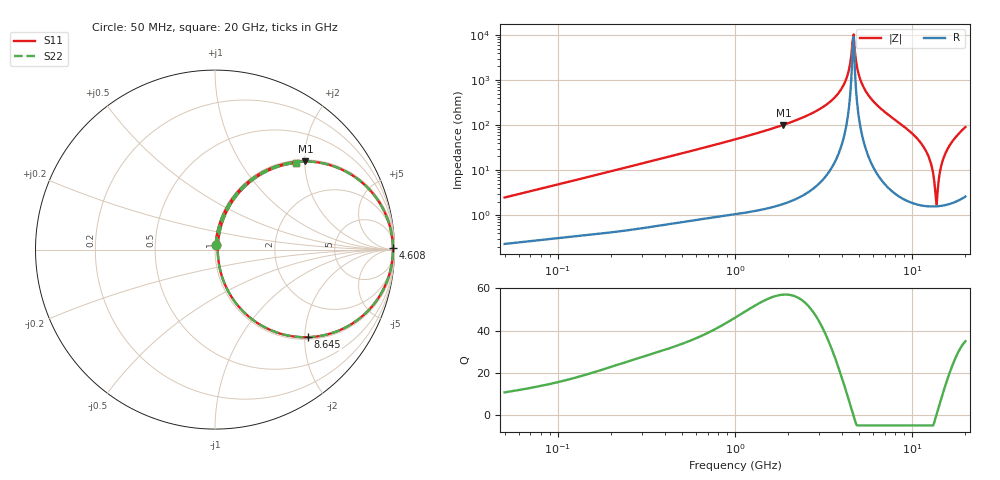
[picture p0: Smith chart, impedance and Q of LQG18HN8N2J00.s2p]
!Murata Part Number: LQG18HN8N2J00
!These Parameters are Measured in Series Mode Connection
!  o--[Z]--o
!Port1  Port2
!  o-------o
!Freq. Start=50[MHz] Stop=20[GHz], 401[Steps]
# Hz S RI R 50
!Freq.(Hz) S11(Real) S11(Imag) S21(Real) S21(Imag) S12(Real) S12(Imag) S22(Real) S22(Imag)
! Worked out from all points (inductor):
!   401 points, 50 MHz to 20 GHz, reference 50 ohm
!   read as one part in series: L = 7.7 nH near 51.52 MHz
!   highest Q = 57.1 at 1.876 GHz (marker M1), where L = 8.55 nH
!   self-resonance near 4.608 GHz
!   S11 on the Smith chart (normalised r, x): 50 MHz: 1.00, +0.05; 4.608 GHz: open; 8.645 GHz: 1.05, -2.08; 20 GHz: 1.05, +1.80
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5e7  0.00287 0.0243  0.9971 -0.0243  0.9971 -0.0243  0.00287 0.0243
1.364002e8  0.0076 0.0639  0.9924 -0.0639  0.9924 -0.0639  0.0076 0.0639
3.721004e8  0.0347 0.1672  0.9653 -0.1672  0.9653 -0.1672  0.0347 0.1672
1e9  0.1919 0.3831  0.8081 -0.3831  0.8081 -0.3831  0.1919 0.3831
1.875929e9  0.5037 0.4913  0.4963 -0.4913  0.4963 -0.4913  0.5037 0.4913
2.728004e9  0.7661 0.4133  0.2339 -0.4133  0.2339 -0.4133  0.7661 0.4133
3.415248e9  0.904 0.2802  0.096 -0.2802  0.096 -0.2802  0.904 0.2802
3.967106e9  0.9662 0.1562  0.0338 -0.1562  0.0338 -0.1562  0.9662 0.1562
4.34015e9  0.9864 0.071  0.0136 -0.071  0.0136 -0.071  0.9864 0.071
4.608136e9  0.9914 0.0108  0.00861 -0.0108  0.00861 -0.0108  0.9914 0.0108
4.748272e9  0.9911 -0.02  0.00895 0.02  0.00895 0.02  0.9911 -0.02
5.041459e9  0.9844 -0.0824  0.0156 0.0824  0.0156 0.0824  0.9844 -0.0824
5.433528e9  0.9641 -0.1608  0.0359 0.1608  0.0359 0.1608  0.9641 -0.1608
7.442007e9  0.7197 -0.4376  0.2803 0.4376  0.2803 0.4376  0.7197 -0.4376
8.644534e9  0.5194 -0.4881  0.4806 0.4881  0.4806 0.4881  0.5194 -0.4881
1.183995e10  0.0888 -0.2583  0.9112 0.2583  0.9112 0.2583  0.0888 -0.2583
1.276073e10  0.034 -0.1344  0.966 0.1344  0.966 0.1344  0.034 -0.1344
1.334722e10  0.0181 -0.0524  0.9819 0.0524  0.9819 0.0524  0.0181 -0.0524
1.375312e10  0.0154 0.00387  0.9846 -0.00387  0.9846 -0.00387  0.0154 0.00387
1.482269e10  0.0375 0.1443  0.9625 -0.1443  0.9625 -0.1443  0.0375 0.1443
1.573793e10  0.0844 0.2489  0.9156 -0.2489  0.9156 -0.2489  0.0844 0.2489
2e10  0.4499 0.4834  0.5501 -0.4834  0.5501 -0.4834  0.4499 0.4834
